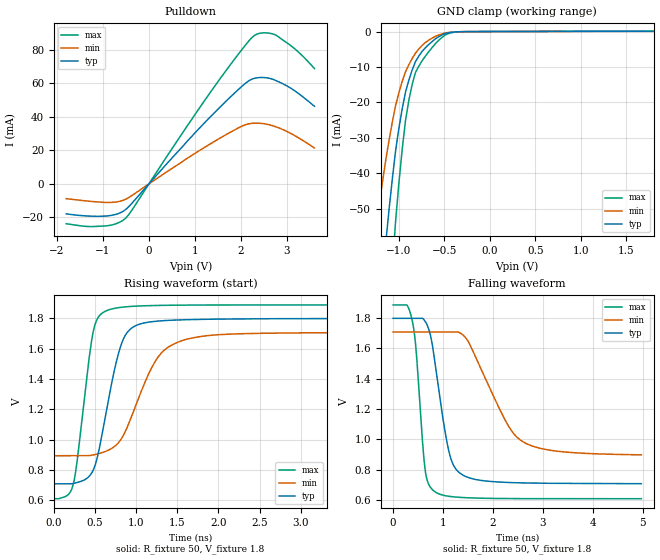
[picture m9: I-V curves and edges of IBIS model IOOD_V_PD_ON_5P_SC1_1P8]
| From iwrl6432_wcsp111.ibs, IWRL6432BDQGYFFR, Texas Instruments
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|   Model Cell IOOD_V_PD_ON_5P_SC1_1P8
|IOOD_V_PD_ON_5P_SC1_1P8
[Model]   IOOD_V_PD_ON_5P_SC1_1P8
Model_type   I/O_open_drain
Polarity   Non-Inverting
Enable   Active-Low
Vinl =  0.63
Vinh =  1.17
Cref =  15pF
Rref =  100.0000M
Vref =  0V
Vmeas =  0.9
|   typ   min   max
C_comp   2.233931p   2.204415p   2.290246p
[Model Spec]
Vinl   0.63   0.5985   0.6615
Vinh   1.17   1.1115   1.2285
[Temperature Range]   25   125   -40
[Voltage Range]   1.8   1.71   1.89
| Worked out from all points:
|   slope of the pulldown table from 0 to 0.27 V, typ, clamps not added: 32.2 ohm
|   GND clamp passes 1 mA (typ) near -0.53 V on its own axis
|   rising waveform, R_fixture 50, V_fixture 1.8: 20-80 % time 246ps typ, 396ps min, 169ps max; typ from 0.708 V to 1.8 V
|   falling waveform, R_fixture 50, V_fixture 1.8: 20-80 % time 308ps typ, 717ps min, 171ps max; typ from 1.8 V to 0.708 V
| Where Nom  PVT is Nominal Process, 1.8V, 25C
|   Fast PVT is Strong Process,  1.89V, -40C
|   Slow PVT is Weak Process,   1.71V, 125C
[Pulldown]
|   voltage   I(typ)   I(min)   I(max)
-1.8V     -17.92mA   -8.85mA    -23.8mA
-1.309V   -19.26mA   -10.37mA   -25.5mA
-927.3mV  -19.22mA   -11.12mA   -25.08mA
-654.5mV  -17.65mA   -10.56mA   -23.13mA
-490.9mV  -14.97mA   -8.985mA   -20.05mA
1.364V    40.78mA    24.32mA    55.69mA
2.073V    59.4mA     35mA       81.9mA
2.291V    62.96mA    36.2mA     88.48mA
2.509V    63.41mA    35.84mA    90.12mA
2.782V    61.38mA    33.82mA    88.42mA
3.218V    54.59mA    28.02mA    79.45mA
3.6V      46.26mA    21.39mA    68.79mA
[GND_clamp]
|   voltage   I(typ)   I(min)   I(max)
-1.8V     -270.2mA   -170.2mA   -430.1mA
-1.255V   -91.66mA   -55.91mA   -148.4mA
-1.145V   -59.91mA   -36.45mA   -97.1mA
-1.109V   -50.48mA   -30.83mA   -81.56mA
-1.073V   -41.73mA   -25.65mA   -67.06mA
-1.036V   -33.67mA   -20.93mA   -53.6mA
-927.3mV  -17.08mA   -11.35mA   -25.06mA
-854.5mV  -10.88mA   -7.624mA   -14.94mA
-781.8mV  -6.944mA   -4.956mA   -9.81mA
-636.4mV  -2.852mA   -1.883mA   -4.567mA
-381.8mV  -107.5uA   -92.09uA   -158.2uA
1.8V      101.9uA    59.12uA    150.8uA
[Ramp]
| variable   typ   min   max
dV/dt_f 0.66096344/0.31032057n 0.49614538/0.73309515n 0.77261485/0.17237057n
dV/dt_r 0.65867605/0.43206823n 0.50260003/0.96153533n 0.77694652/0.24600924n
R_load = 50
[Rising Waveform]
R_fixture = 50
V_fixture = 1.8
V_fixture_min = 1.71
V_fixture_max = 1.89
|   time   V(typ)   V(min)   V(max)
0s        708.5mV    893.6mV    610.5mV
234.6ps   710.6mV    893.6mV    702.7mV
472.3ps   792.1mV    898mV      1.694V
530.6ps   888.5mV    905.2mV    1.798V
629.5ps   1.163V     922.2mV    1.847V
776.9ps   1.55V      974.4mV    1.869V
898.1ps   1.71V      1.09V      1.876V
1.247ns   1.78V      1.528V     1.884V
1.557ns   1.789V     1.652V     1.886V
4.974ns   1.798V     1.707V     1.887V
[Falling Waveform]
R_fixture = 50
V_fixture = 1.8
V_fixture_min = 1.71
V_fixture_max = 1.89
|   time   V(typ)   V(min)   V(max)
0s        1.798V     1.708V     1.887V
275ps     1.798V     1.708V     1.887V
378.3ps   1.798V     1.708V     1.79V
458.2ps   1.798V     1.708V     1.598V
639.1ps   1.78V      1.708V     806.6mV
815.9ps   1.559V     1.708V     660.4mV
1.117ns   921.1mV    1.708V     624.7mV
1.373ns   769.9mV    1.695V     617.2mV
2.561ns   713.4mV    993.5mV    609.5mV
4.974ns   708mV      898.7mV    609.1mV
